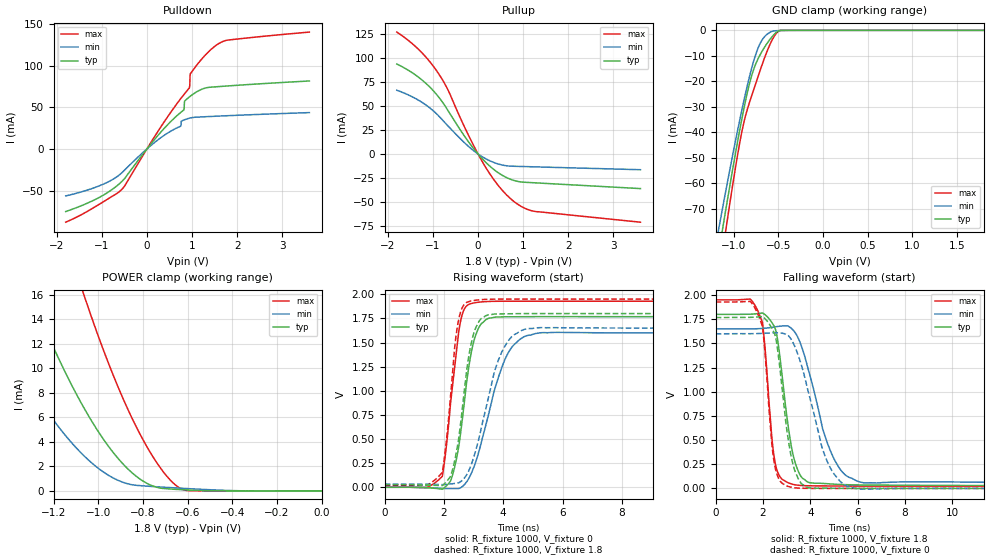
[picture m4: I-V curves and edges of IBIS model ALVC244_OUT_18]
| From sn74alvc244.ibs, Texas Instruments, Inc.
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[Model]   ALVC244_OUT_18
Model_type  3-state
Enable   Active-Low
Vref =   0
Rref =   1000
Cref =   30p
Vmeas =   0.9
| variable   typ   min   max
C_comp   6.53pF   5.75pF   7.29pF
| C_pullup   8.80pF   6.36pF   10.24pF
| C_pulldown   16.66pF   6.55pF   36.00pF
| C_tri-state   6.53pF   5.75pF   7.29pF
[Temperature Range]   40   100   -40
| Ambient temperature   25   85   -40
[Voltage range]   1.8   1.65   1.95
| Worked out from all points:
|   slope of the pulldown table from 0 to 0.27 V, typ, clamps not added: 15.1 ohm
|   slope of the pullup table from 0 to 0.27 V, typ, clamps not added: 20.7 ohm
|   GND clamp passes 1 mA (typ) near -0.53 V on its own axis
|   POWER clamp passes 1 mA (typ) near -0.82 V on its own axis
|   rising waveform, R_fixture 1000, V_fixture 0: 20-80 % time 474ps typ, 869ps min, 406ps max; typ from 0 V to 1.77 V
|   falling waveform, R_fixture 1000, V_fixture 1.8: 20-80 % time 573ps typ, 1.1ns min, 384ps max; typ from 1.8 V to 0.026 V
|   rising waveform, R_fixture 1000, V_fixture 1.8: 20-80 % time 460ps typ, 799ps min, 351ps max; typ from 0.026 V to 1.8 V
|   falling waveform, R_fixture 1000, V_fixture 0: 20-80 % time 544ps typ, 1.03ns min, 374ps max; typ from 1.77 V to 0 V
[GND Clamp]
| ALVC244_OUT_18
|   Voltage   I(typ)   I(min)   I(max)
-1.8V     -231.2mA   -205.8mA   -257.4mA
-1.175V   -88.93mA   -79.43mA   -99.17mA
-1.15V    -83.55mA   -74.67mA   -93.15mA
-1.11V    -75.03mA   -67.13mA   -83.61mA
-1.09V    -70.82mA   -63.4mA    -78.9mA
-1.07V    -66.64mA   -59.7mA    -74.23mA
-915mV    -36.06mA   -32.44mA   -41.08mA
-820mV    -20.6mA    -17.82mA   -28.03mA
-715mV    -10.36mA   -6.036mA   -16.97mA
-595mV    -3.622mA   -819.5uA   -5.693mA
-475mV    -33.84uA   -89.41uA   -29.91uA
1.8V      72.03pA    22.9nA     9.218pA
[POWER Clamp]
| ALVC244_OUT_18
|   Voltage   I(typ)   I(min)   I(max)
-1.8V     42.94mA    26.89mA    69.48mA
-1.53V    27.31mA    16.02mA    47.28mA
-1.3V     15.93mA    8.44mA     30.5mA
-1.18V    10.9mA     5.281mA    22.73mA
-1.06V    6.645mA    2.798mA    15.77mA
-990mV    4.572mA    1.715mA    12.14mA
-915mV    2.735mA    896.2uA    8.646mA
-835mV    1.271mA    466.8uA    5.424mA
-755mV    395.8uA    357.4uA    2.787mA
-685mV    167uA      278.6uA    1.038mA
-630mV    105uA      220.7uA    191.4uA
-16.28fV  72.03pA    466pA      10.31pA
[Pulldown]
| ALVC244_OUT_18
|   Voltage   I(typ)   I(min)   I(max)
-1.8V     -75.32mA   -56.53mA   -88.08mA
-970mV    -55.69mA   -42.44mA   -63.7mA
-525mV    -37.45mA   -27.03mA   -46.75mA
270mV     17.84mA    11.99mA    23.28mA
820mV     46.98mA    34.77mA    65.34mA
835mV     57.53mA    35.09mA    66.37mA
940mV     62.45mA    36.95mA    73.27mA
950mV     62.89mA    37.08mA    75.97mA
960mV     63.31mA    37.21mA    90.13mA
1.495V    74.54mA    39.22mA    123mA
1.785V    75.69mA    39.93mA    130.8mA
3.6V      81.68mA    43.67mA    140.4mA
[Pullup]
| ALVC244_OUT_18
|   Voltage   I(typ)   I(min)   I(max)
-1.8V     93.89mA    66.52mA    127.2mA
-1.315V   79.96mA    56mA       109mA
-1.105V   71.48mA    49.38mA    98.38mA
-915mV    61.88mA    41.72mA    86.66mA
-680mV    46.35mA    29.97mA    68.15mA
-240mV    14.57mA    9.093mA    22.28mA
125mV     -6.524mA   -3.765mA   -10.47mA
460mV     -19.97mA   -10.61mA   -33.57mA
800mV     -27.68mA   -12.83mA   -49.74mA
1.03V     -29.51mA   -13.14mA   -56.52mA
1.26V     -30.1mA    -13.44mA   -59.95mA
3.6V      -36.12mA   -16.42mA   -71.2mA
[Ramp]
| ALVC244_OUT_18
| variable   typ   min   max
dV/dt_r   1.07/4.97E-10   0.97/9.04E-10   1.16/4.28E-10
dV/dt_f   1.07/5.94E-10   0.99/1.19E-09   1.16/4.08E-10
R_load = 1000
[Rising Waveform]
| ALVC244_OUT_18
R_fixture =   1000
C_fixture =   0
L_fixture =   0
V_fixture =   0
V_fixture_min = 0
V_fixture_max = 0
|   Time   V(typ)   V(min)   V(max)
0s        50.9pV     4.429nV    37.8pV
1.945ns   -19.62mV   -12.18mV   113.1mV
2.225ns   66.19mV    -13.83mV   876mV
2.5ns     421.3mV    -13.24mV   1.613V
2.605ns   664.3mV    4.096mV    1.776V
2.885ns   1.334V     119.2mV    1.901V
3.16ns    1.644V     349.6mV    1.917V
4.13ns    1.767V     1.371V     1.928V
5.265ns   1.768V     1.601V     1.928V
50ns      1.768V     1.6V       1.928V
[Falling Waveform]
| ALVC244_OUT_18
R_fixture =   1000
C_fixture =   0
L_fixture =   0
V_fixture =   1.8
V_fixture_min = 1.65
V_fixture_max = 1.95
|   Time   V(typ)   V(min)   V(max)
0s        1.8V       1.65V      1.95V
1.455ns   1.801V     1.649V     1.958V
1.93ns    1.812V     1.653V     1.745V
2.5ns     1.665V     1.67V      280mV
3.12ns    548.4mV    1.67V      52.83mV
3.39ns    242.3mV    1.599V     36.05mV
3.89ns    66.31mV    1.25V      27.65mV
4.925ns   45.48mV    344.9mV    25.32mV
6.245ns   35.68mV    58.54mV    24.3mV
50ns      25.63mV    35.26mV    21.74mV
[Rising Waveform]
| ALVC244_OUT_18
R_fixture =   1000
C_fixture =   0
L_fixture =   0
V_fixture =   1.8
V_fixture_min = 1.65
V_fixture_max = 1.95
|   Time   V(typ)   V(min)   V(max)
0s        25.6mV     33.9mV     21.73mV
1.945ns   17.66mV    27.43mV    154mV
2.22ns    113mV      33.98mV    933.1mV
2.38ns    301.7mV    40.45mV    1.498V
2.54ns    604.7mV    53.6mV     1.792V
2.835ns   1.353V     168.8mV    1.923V
3.11ns    1.675V     422.1mV    1.94V
3.985ns   1.797V     1.423V     1.95V
5.145ns   1.8V       1.653V     1.95V
50ns      1.8V       1.65V      1.95V
[Falling Waveform]
| ALVC244_OUT_18
R_fixture =   1000
C_fixture =   0
L_fixture =   0
V_fixture =   0
V_fixture_min = 0
V_fixture_max = 0
|   Time   V(typ)   V(min)   V(max)
0s        1.768V     1.6V       1.928V
1.455ns   1.769V     1.6V       1.934V
1.855ns   1.774V     1.603V     1.758V
2.015ns   1.77V      1.604V     1.585V
2.4ns     1.643V     1.608V     396.3mV
2.685ns   1.3V       1.609V     91.23mV
3.27ns    244mV      1.506V     9.093mV
4.73ns    2.711mV    269.7mV    78.14uV
6.015ns   260.7uV    -5.282mV   181uV
50ns      2.859uV    43.5uV     356nV
